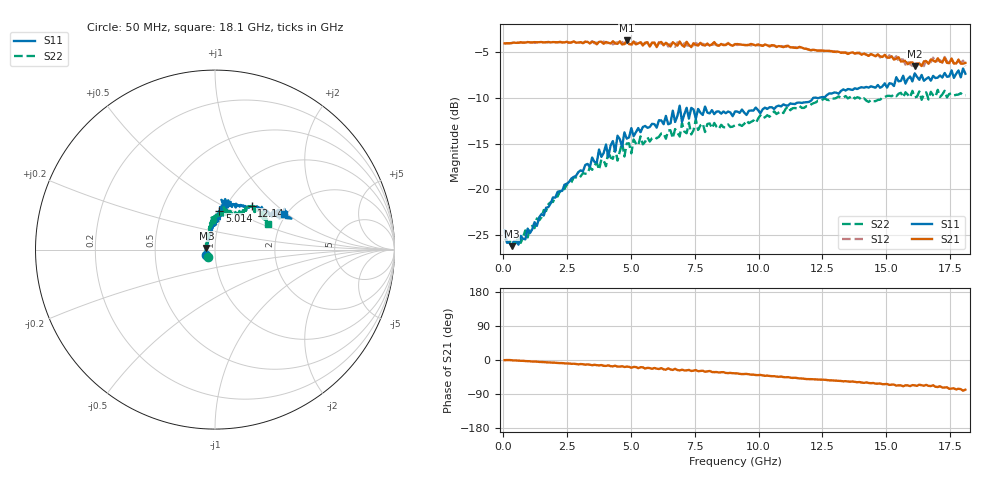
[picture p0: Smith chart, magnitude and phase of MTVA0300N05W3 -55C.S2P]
! Network Analyzer HP8720D.06.14 Serial No. US36140669
!  7 Jul 2005  09:13:12
! Frequency  S11  S21  S12  S22
# HZ  S  DB R 50
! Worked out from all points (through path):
!   201 points, 50 MHz to 18.1 GHz, reference 50 ohm
!   highest |S21| = -3.68 dB at 4.833 GHz (marker M1); lowest = -6.5 dB at 16.11 GHz (marker M2)
!   group delay of S21, straight-line fit = 12.1 ps
!   lowest |S11| = -26.2 dB at 320.8 MHz (marker M3), VSWR 1.10, Z = 45.4 + j0.872 ohm
!   |S11| at or under -10 dB: start of sweep to 12.13 GHz; 12.30466 GHz to 12.33909 GHz (34.43 MHz wide, 0.279 % of centre)
!   |S22| runs from -25.9 to -9.1 dB; largest |S21 - S12| = 0.04
!   S11 on the Smith chart (normalised r, x): 50 MHz: 0.90, -0.06; 5.014 GHz: 0.95, +0.43; 12.14 GHz: 1.30, +0.70; 18.1 GHz: 1.94, +0.94
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5e7  -24.49 -148.1  -4.00 -0.4  -4.02 -0.1  -25.40 -134.2
3.2075e8  -26.23 168.7  -3.97 -0.7  -3.97 -0.8  -25.47 170.1
9.525e8  -24.30 136.4  -3.86 -3.0  -3.90 -2.9  -25.27 141.8
3.1185e9  -18.03 95.5  -3.97 -11.1  -3.98 -11.6  -18.23 105.7
4.382e9  -15.87 85.9  -4.01 -15.1  -3.93 -17.1  -15.39 95.8
4.47225e9  -14.12 80.9  -4.05 -17.4  -3.89 -15.6  -16.84 99.6
4.65275e9  -15.31 80.9  -4.12 -16.4  -3.84 -17.9  -14.87 97.5
4.743e9  -13.76 83.2  -4.08 -18.4  -4.05 -16.9  -16.40 93.7
4.83325e9  -14.44 88.7  -3.68 -17.6  -3.96 -19.2  -14.98 86.6
5.01375e9  -13.29 83.6  -4.11 -20.4  -4.21 -18.6  -16.05 89.0
5.104e9  -14.18 85.2  -3.81 -18.4  -3.90 -19.8  -14.53 88.4
6.09675e9  -12.43 78.4  -3.94 -23.7  -3.87 -23.2  -14.24 84.0
6.7285e9  -12.62 83.0  -4.06 -23.3  -4.38 -24.8  -13.39 76.6
6.909e9  -10.83 78.7  -3.80 -27.7  -4.01 -25.5  -14.21 76.3
6.99925e9  -12.61 78.7  -4.19 -25.4  -4.32 -28.1  -12.74 76.1
7.17975e9  -11.06 82.7  -3.83 -27.4  -4.23 -26.1  -13.85 71.5
7.54075e9  -12.26 73.7  -4.16 -26.5  -3.95 -29.9  -12.36 78.3
9.075e9  -11.47 71.9  -4.10 -35.1  -4.06 -35.1  -12.98 65.4
1.21435e10  -9.97 50.0  -4.70 -50.7  -4.65 -50.7  -10.56 53.1
1.512175e10  -8.38 29.5  -5.58 -65.7  -5.30 -65.2  -9.75 40.7
1.61145e10  -7.29 27.7  -6.52 -66.9  -5.99 -66.9  -9.92 37.2
1.81e10  -7.33 27.3  -6.15 -78.3  -6.50 -78.2  -9.69 25.3
